(* Logix 5000 AddOnInstructionDefinition export Banner_S15C_MUL_PD_v2; software revision 32.00 *)

TYPE Banner_S15C_MUL_PDIO_v2 :   // UDT with all of the variables needed to control an IO-Link S15C UL.
STRUCT
   Distance_mm : REAL;
   Distance_in : REAL;
   Temperature_C : REAL;
   Temperature_F : REAL;
   DTI : SINT[8];   // Array with Raw Process data being transferred into AOI.
END_STRUCT
END_TYPE

ADD_ON_INSTRUCTION Banner_S15C_MUL_PD_v2   (* revision 2.0, vendor Banner Engineering *)
// AOI that used with the S15C MUL sensor.
VAR_IN_OUT
   Process_Data : Banner_S15C_MUL_PDIO_v2; {required}
END_VAR
VAR_INPUT
   Byte_Swap : BOOL; {required}
END_VAR
VAR
   Temp_DWord : DINT[4]; {access None}
END_VAR

ROUTINE Logic   (* ladder *)
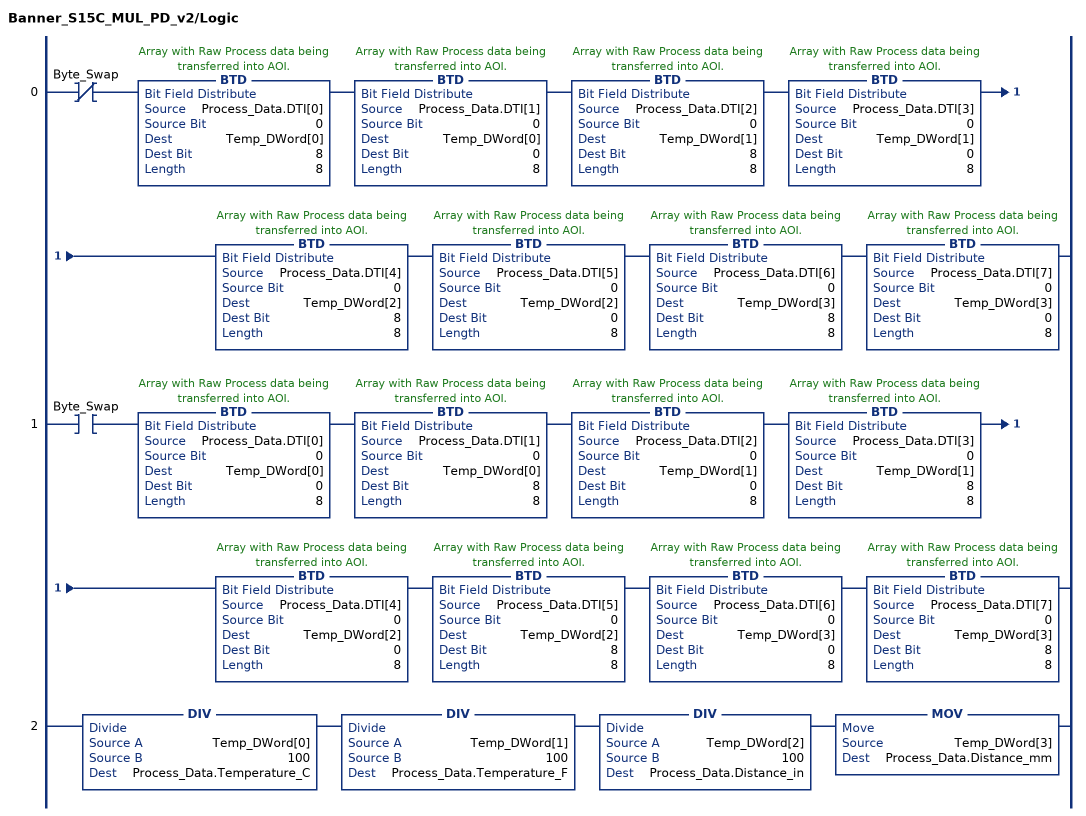
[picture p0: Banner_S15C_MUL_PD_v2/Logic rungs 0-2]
   0: XIO(Byte_Swap)BTD(Process_Data.DTI[0],0,Temp_DWord[0],8,8)BTD(Process_Data.DTI[1],0,Temp_DWord[0],0,8)BTD(Process_Data.DTI[2],0,Temp_DWord[1],8,8)BTD(Process_Data.DTI[3],0,Temp_DWord[1],0,8)BTD(Process_Data.DTI[4],0,Temp_DWord[2],8,8)BTD(Process_Data.DTI[5],0,Temp_DWord[2],0,8)BTD(Process_Data.DTI[6],0,Temp_DWord[3],8,8)BTD(Process_Data.DTI[7],0,Temp_DWord[3],0,8);
   1: XIC(Byte_Swap)BTD(Process_Data.DTI[0],0,Temp_DWord[0],0,8)BTD(Process_Data.DTI[1],0,Temp_DWord[0],8,8)BTD(Process_Data.DTI[2],0,Temp_DWord[1],0,8)BTD(Process_Data.DTI[3],0,Temp_DWord[1],8,8)BTD(Process_Data.DTI[4],0,Temp_DWord[2],0,8)BTD(Process_Data.DTI[5],0,Temp_DWord[2],8,8)BTD(Process_Data.DTI[6],0,Temp_DWord[3],0,8)BTD(Process_Data.DTI[7],0,Temp_DWord[3],8,8);
   2: DIV(Temp_DWord[0],100,Process_Data.Temperature_C)DIV(Temp_DWord[1],100,Process_Data.Temperature_F)DIV(Temp_DWord[2],100,Process_Data.Distance_in)MOV(Temp_DWord[3],Process_Data.Distance_mm);
END_ROUTINE
END_ADD_ON_INSTRUCTION
